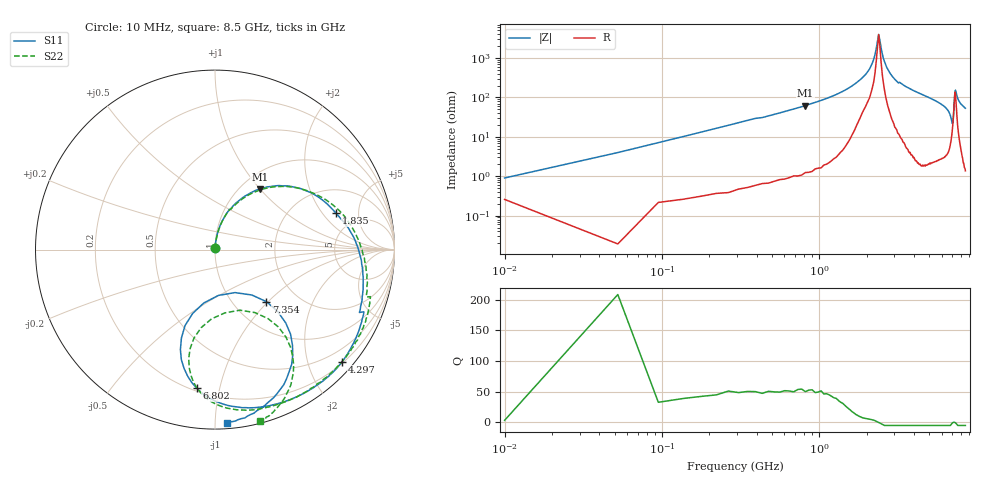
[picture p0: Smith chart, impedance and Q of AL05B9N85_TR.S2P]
!AVX Corporation
!PN: AL05B9N85*TR
!Description: Air Core Inductor, 9.85nH, 9 Turns
!Agilent Technologies,E5071C,MY46102230,A.09.54
!Date: Mon Sep 03 16:23:13 2012
!Data & Calibration Information:
!Freq	S11:SOLT2(ON)	S21:SOLT2(ON)	S12:SOLT2(ON)	S22:SOLT2(ON)
# Hz S dB R 50
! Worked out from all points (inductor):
!   201 points, 10 MHz to 8.5 GHz, reference 50 ohm
!   read as 1/Y11, port 2 shorted: L = 11.9 nH near 52.45 MHz
!   highest Q = 53.1 at 816.5 MHz (marker M1), where L = 12.1 nH
!   self-resonance near 2.387 GHz
!   S11 on the Smith chart (normalised r, x): 10 MHz: 1.00, +0.01; 1.835 GHz: 3.44, +2.77; 4.297 GHz: 0.23, -2.62; 6.802 GHz: 0.22, -0.85; 7.354 GHz: 1.41, -0.98; 8.5 GHz: 0.04, -1.07
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1e7  -43.26 79.9  -0.01 -0.5  -0.06 -0.7  -43.25 79.7
5.245e7  -29.37 85.4  -0.02 -2.6  0.03 -2.7  -29.35 85.0
9.49e7  -24.41 83.3  -0.04 -4.6  -0.03 -4.7  -24.37 82.8
1.798e8  -18.98 79.7  -0.08 -8.7  -0.07 -8.7  -18.91 79.4
3.9205e8  -12.53 70.3  -0.30 -18.6  -0.29 -18.6  -12.50 69.9
8.1655e8  -7.55 53.5  -0.94 -35.8  -0.93 -35.8  -7.55 52.7
1.4533e9  -4.02 29.5  -2.42 -59.9  -2.42 -59.9  -3.97 29.6
1.83535e9  -3.03 16.7  -3.52 -72.5  -3.52 -72.6  -2.80 17.7
2.85415e9  -1.39 -14.3  -6.30 -100.9  -6.30 -100.9  -1.32 -9.5
4.255e9  -0.51 -40.8  -10.56 -126.8  -10.57 -126.9  -0.53 -35.6
4.29745e9  -0.50 -41.5  -10.63 -127.6  -10.63 -127.6  -0.52 -36.4
5.6983e9  -0.61 -65.3  -11.30 -155.4  -11.29 -155.4  -0.60 -65.8
6.4624e9  -1.14 -84.0  -9.19 -176.5  -9.19 -176.5  -1.00 -84.5
6.802e9  -2.18 -97.6  -6.74 165.8  -6.75 165.8  -1.94 -95.8
6.9718e9  -3.86 -107.0  -5.11 150.1  -5.11 150.1  -3.42 -102.3
7.09915e9  -6.85 -111.5  -3.96 132.9  -3.96 132.9  -5.90 -103.4
7.2265e9  -11.84 -85.8  -3.51 110.0  -3.51 110.0  -8.95 -81.1
7.26895e9  -11.56 -65.0  -3.64 101.4  -3.65 101.4  -8.75 -67.6
7.35385e9  -7.80 -45.3  -4.37 85.3  -4.37 85.2  -6.27 -52.4
7.52365e9  -3.27 -51.0  -7.04 60.1  -7.04 60.1  -2.67 -54.0
7.77835e9  -1.31 -65.0  -11.25 39.1  -11.26 39.0  -0.95 -63.5
8.5e9  -0.29 -86.1  -18.99 14.4  -18.99 14.3  -0.11 -75.2
